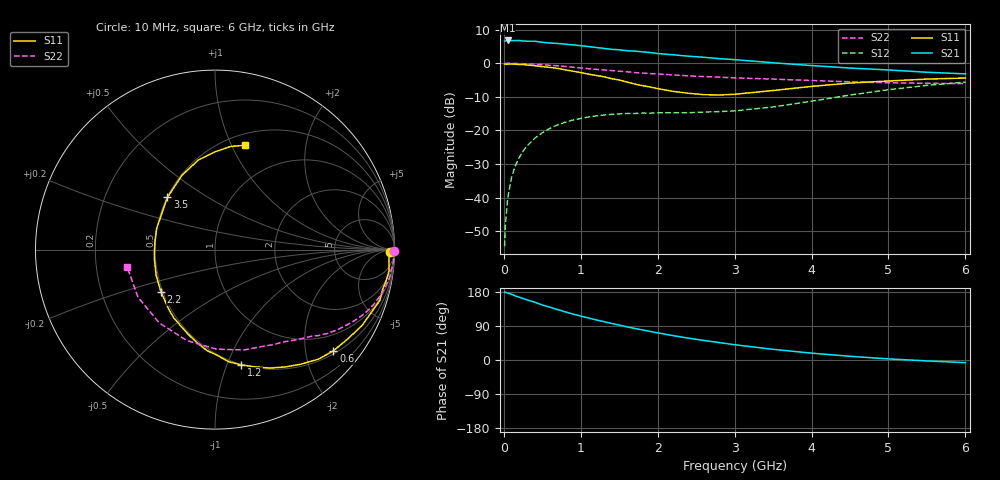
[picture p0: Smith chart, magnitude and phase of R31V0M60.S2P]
! SIEMENS Small Signal Semiconductors
! BFR181
! Si NPN RF Bipolar Junction Transistor in SOT23
! VCE = 1 V  IC = 0.6 mA
! Common Emitter S-Parameters:  May  1996
# GHz  S  MA  R  50
!  f  S11  S21  S12  S22
! GHz  MAG  ANG  MAG  ANG  MAG  ANG  MAG  ANG
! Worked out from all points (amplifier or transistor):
!   36 points, 10 MHz to 6 GHz, reference 50 ohm
!   highest |S21| = 6.8 dB at 50 MHz (marker M1)
!   |S21| within 3 dB of that: start of sweep to 1.579 GHz
!   unconditionally stable (mu >= 1): 2.198 GHz to 4.115 GHz
!   at 250 MHz: K = 0.13, MSG = 16.4 dB, |S12| = -26.1 dB
!   at 1.4 GHz: K = 0.67, MSG = 9.7 dB, |S12| = -15.2 dB
!   at 6 GHz: K = 0.95, MSG = 1.2 dB, |S12| = -5.6 dB
!   S11 on the Smith chart (normalised r, x): 10 MHz: 64, -31; 600 MHz: 0.57, -2.60; 1.2 GHz: 0.50, -1.13; 2.2 GHz: 0.49, -0.27; 3.5 GHz: 0.50, +0.35; 6 GHz: 0.62, +1.13
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0.01  0.9749 -0.7  2.152 179.7  0.0019 90.2  0.9984 -0.4
0.02  0.9705 -1.1  2.146 178.6  0.0039 88.4  0.9942 -0.7
0.05  0.971 -3.6  2.187 176.8  0.0099 87.5  0.9984 -1.7
0.1  0.9769 -6.9  2.174 173.4  0.0201 86.0  0.9968 -3.3
0.15  0.9695 -10.3  2.18 169.1  0.0299 82.1  0.9937 -5.1
0.25  0.9611 -17.1  2.147 162.4  0.0494 77.8  0.9865 -8.5
0.4  0.922 -27.3  2.128 152.6  0.0765 71.5  0.9682 -13.2
0.5  0.8913 -34.0  2.056 145.2  0.0925 67.0  0.9516 -16.3
0.6  0.8678 -40.5  2.001 139.2  0.1079 62.8  0.935 -19.1
0.7  0.84 -46.6  1.974 133.1  0.1214 59.1  0.9162 -21.8
0.9  0.7625 -59.0  1.88 121.1  0.1433 52.0  0.8738 -26.8
1.1  0.69 -71.2  1.776 110.9  0.1585 46.2  0.8325 -31.2
1.2  0.6591 -77.1  1.716 105.8  0.1651 43.4  0.8141 -33.4
1.4  0.5909 -88.5  1.612 96.5  0.1736 39.1  0.7798 -36.9
1.7  0.4916 -108.3  1.519 83.4  0.179 35.3  0.7278 -41.3
2.2  0.3823 -142.0  1.338 64.3  0.1831 32.7  0.6716 -48.7
2.6  0.3413 -172.5  1.228 51.6  0.1878 34.9  0.6344 -54.6
2.8  0.3375 173.8  1.173 46.0  0.1912 36.6  0.6225 -58.3
3.5  0.3937 132.3  1.019 28.2  0.224 43.3  0.5819 -73.9
4.5  0.5081 100.5  0.85 9.8  0.337 44.1  0.5305 -107.3
5.5  0.5819 81.2  0.736 -2.4  0.4694 32.1  0.5043 -148.3
6  0.6041 74.0  0.696 -7.0  0.5251 23.8  0.4991 -168.8
